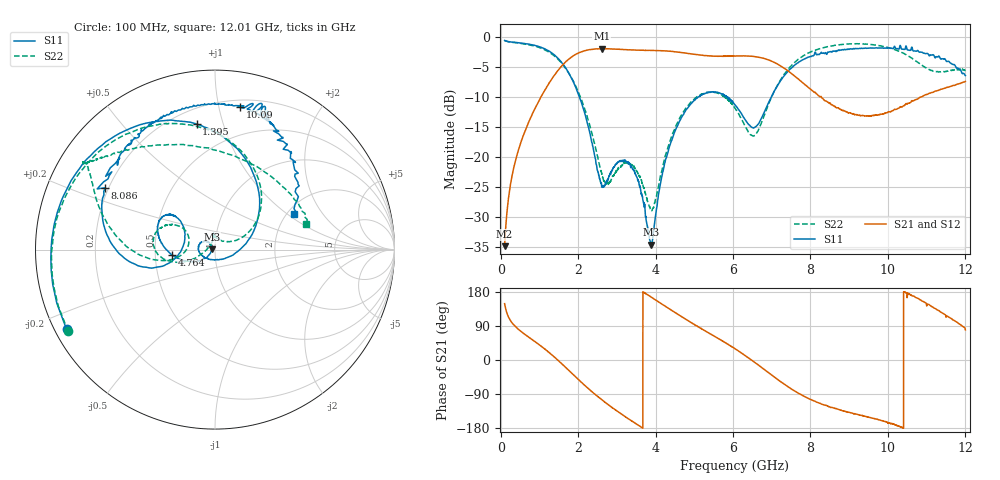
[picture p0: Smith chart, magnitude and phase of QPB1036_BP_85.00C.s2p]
! TDS: K:\Engsetup\Winsaw\QPB1036_ALL
! Channel 1
! Ports=1 2
! seg 1=100.000000 1100.000000 101
! seg 2=1101.000000 1501.000000 401
! seg 3=1502.000000 2502.000000 101
! seg 4=2503.000000 3803.000000 1301
! seg 5=3804.000000 5004.000000 121
! seg 6=5005.000000 6005.000000 1001
! seg 7=6006.000000 8406.000000 241
! seg 8=8407.000000 10607.000000 2201
! seg 9=10608.000000 12008.000000 141
! Points=5609
! FailCode=0
! Topology=ALL_SE(12)
!VNA Cal loaded =QPB1036_ALL_85C
!PS1(V)= 5.000
!PS(mA)= 0.700
!PS2(V)= 1.170
!PS(mA)= -0.100
!PS3(V)= 1.170
!PS(mA)= 0.100
!PS4(V)= 1.170
!PS(mA)= -0.100
!Temp (C)= 85.00
# MHz S DB R 50
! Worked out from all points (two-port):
!   5609 points, 100 MHz to 12.01 GHz, reference 50 ohm
!   highest |S21| = -1.92 dB at 2.61 GHz (marker M1); lowest = -34.9 dB at 100 MHz (marker M2)
!   |S21| within 3 dB of the highest: 1.562 GHz to 7.262 GHz (5.7 GHz wide, 129 % of centre)
!   lowest |S11| = -34.6 dB at 3.894 GHz (marker M3), VSWR 1.04, Z = 48.2 + j0.115 ohm
!   |S11| at or under -10 dB: 2.036 GHz to 5.101 GHz (3.065 GHz wide, 85.9 % of centre); 5.858843 GHz to 5.86185 GHz (3.007 MHz wide, 0.0513 % of centre); 5.862 GHz to 6.99 GHz (1.128 GHz wide, 17.6 % of centre)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
!   |S22| runs from -29.0 to -0.6 dB; largest |S21 - S12| = 0.11
!   S11 on the Smith chart (normalised r, x): 100 MHz: 0.03, -0.25; 1.395 GHz: 0.29, +0.82; 4.764 GHz: 0.62, -0.04; 8.086 GHz: 0.19, +0.25; 10.09 GHz: 0.25, +1.16; 12.01 GHz: 2.16, +1.10
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100  -0.55 -151.8  -34.86 148.6  -34.83 148.8  -0.57 -151.0
720  -1.16 145.4  -14.21 60.5  -14.19 60.3  -1.26 149.0
1395  -3.02 98.4  -6.29 7.1  -6.28 6.9  -3.19 98.2
2092  -11.05 33.6  -2.41 -59.7  -2.42 -59.7  -10.53 36.4
2610  -24.99 -75.6  -1.92 -104.6  -1.93 -105.2  -22.68 38.8
3308  -21.09 154.7  -2.11 -155.8  -2.11 -155.9  -21.08 94.4
3792  -31.60 134.7  -2.20 172.2  -2.20 172.1  -27.33 113.7
3894  -34.61 176.3  -2.22 165.5  -2.19 165.3  -28.88 142.6
4074  -26.35 -137.6  -2.25 153.5  -2.23 153.3  -25.00 -171.7
4764  -12.42 -172.6  -2.64 108.6  -2.63 108.2  -12.03 -164.6
5459  -9.13 153.5  -3.16 66.4  -3.12 66.2  -9.18 169.5
6056  -11.31 139.9  -3.15 29.6  -3.11 29.1  -11.86 147.8
6566  -15.04 171.4  -3.25 -6.6  -3.23 -6.7  -16.38 173.9
7126  -8.36 -164.6  -4.40 -49.1  -4.40 -49.5  -8.32 -173.3
8046  -3.12 152.7  -8.91 -105.9  -8.88 -106.4  -2.35 153.0
8086  -3.08 150.6  -9.11 -107.9  -9.07 -108.0  -2.27 152.2
8985  -2.00 112.4  -12.65 -138.0  -12.56 -138.0  -1.13 146.3
10024  -1.76 78.7  -12.43 -166.7  -12.50 -164.8  -1.79 140.7
10087  -1.86 80.1  -12.40 -167.8  -12.35 -167.5  -1.87 140.1
10928  -2.68 63.9  -9.75 154.0  -9.79 153.2  -4.89 96.0
11498  -3.83 46.3  -8.48 118.6  -8.47 117.9  -5.71 40.5
12008  -6.41 24.4  -7.39 79.5  -7.44 87.6  -5.51 14.7
